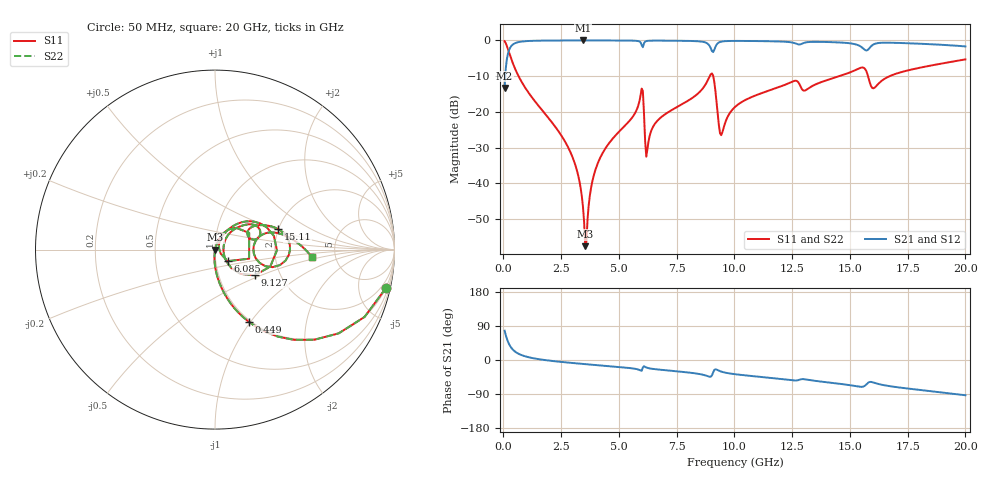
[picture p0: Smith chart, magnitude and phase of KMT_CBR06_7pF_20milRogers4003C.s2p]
! Data measured by Modelithics Inc. support@modelithics.com 813-866-6335
! KEMET CBR0603 7pF, Pad Width= 0.851mm, Pad Length= 0.64mm, Pad Gap= 0.62mm, 20mil Rogers 4003C substrate Data, January 2022
# hz S ma R 50
! 2 Port Network Data from SP1.SP block
! freq  magS11  angS11  magS21  angS21  magS12  angS12  magS22  angS22
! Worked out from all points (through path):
!   401 points, 50 MHz to 20 GHz, reference 50 ohm
!   highest |S21| = -0.01 dB at 3.442 GHz (marker M1); lowest = -13.3 dB at 50 MHz (marker M2)
!   group delay of S21, straight-line fit = 14.1 ps
!   lowest |S11| = -57.6 dB at 3.541 GHz (marker M3), VSWR 1.00, Z = 50.1 - j0.0993 ohm
!   |S11| at or under -10 dB: 654.1 MHz to 8.931 GHz (8.277 GHz wide, 173 % of centre); 9.082 GHz to 14.55 GHz (5.464 GHz wide, 46.2 % of centre); 15.78 GHz to 16.72 GHz (934.8 MHz wide, 5.75 % of centre)
!   |S22| runs from -57.6 to -0.2 dB; largest |S21 - S12| = 0
!   S11 on the Smith chart (normalised r, x): 50 MHz: 0.98, -8.90; 449 MHz: 0.98, -0.98; 6.085 GHz: 1.14, -0.15; 9.127 GHz: 1.49, -0.46; 15.11 GHz: 1.99, +0.53; 20 GHz: 3.32, -0.41
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5e7  0.9762 -12.7  0.2167 77.3  0.2167 77.3  0.9762 -12.7
4.49e8  0.4429 -65.0  0.896 24.9  0.896 24.9  0.4429 -65.0
2.793125e9  0.03231 -95.2  0.9984 -6.8  0.9984 -6.8  0.03231 -95.2
3.391625e9  0.006686 -91.3  0.9988 -10.1  0.9988 -10.1  0.006686 -91.3
3.4415e9  0.004766 -87.9  0.9988 -10.4  0.9988 -10.4  0.004766 -87.9
3.54125e9  0.001324 -48.5  0.9988 -10.9  0.9988 -10.9  0.001324 -48.5
3.890375e9  0.0122 72.0  0.9987 -12.8  0.9987 -12.8  0.0122 72.0
4.289375e9  0.02643 72.6  0.9983 -14.8  0.9983 -14.8  0.02643 72.6
5.93525e9  0.169 45.9  0.9388 -27.7  0.9388 -27.7  0.169 45.9
6.084875e9  0.09495 -42.6  0.9137 -16.4  0.9137 -16.4  0.09495 -42.6
6.2345e9  0.0303 43.5  0.9863 -20.8  0.9863 -20.8  0.0303 43.5
6.73325e9  0.07924 62.5  0.9936 -25.3  0.9936 -25.3  0.07924 62.5
8.778125e9  0.2513 38.9  0.926 -41.3  0.926 -41.3  0.2513 38.9
9.12725e9  0.2645 -32.7  0.7363 -26.4  0.7363 -26.4  0.2645 -32.7
9.4265e9  0.04725 4.7  0.9607 -30.5  0.9607 -30.5  0.04725 4.7
1.0025e10  0.1173 48.2  0.984 -37.5  0.984 -37.5  0.1173 48.2
1.336662e10  0.2297 31.5  0.9549 -54.0  0.9549 -54.0  0.2297 31.5
1.511225e10  0.3691 18.1  0.9011 -67.5  0.9011 -67.5  0.3691 18.1
1.576062e10  0.3361 -16.9  0.7316 -61.4  0.7316 -61.4  0.3361 -16.9
1.601e10  0.2138 0.6  0.8745 -59.2  0.8745 -59.2  0.2138 0.6
1.670825e10  0.3151 17.5  0.9291 -68.9  0.9291 -68.9  0.3151 17.5
2e10  0.5429 -4.6  0.8244 -93.0  0.8244 -93.0  0.5429 -4.6
